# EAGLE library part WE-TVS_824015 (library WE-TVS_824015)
TVS Diode Array WE-TVS, High Speed Series - Low capazity - No leakage current - Low clamping voltage - high ESD voltage protection -- USB 1.0 - 2.0 Double Port -- Ethernet
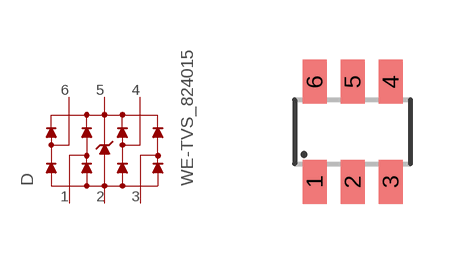
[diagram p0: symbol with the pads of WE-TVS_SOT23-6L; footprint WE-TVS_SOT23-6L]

Designator prefix D

## WE-TVS_824015 (MPN: 824015; OC_FARNELL: 1748615; OC_NEWARK: 34R6122; PACKAGE: SOT23-6L; SUPPLIER: Wuerth Elektronik)  [WE-TVS_SOT23-6L]
1  1  pas
2  GND  pwr
3  2  pas
4  3  pas
5  VDD  pwr
6  4  pas

## Footprint WE-TVS_SOT23-6L (pad centres in mm)
TVS Diode Array WE-TVS
smd 0.6 x 1.1: 1 -0.95,-1.25; 2 0,-1.25; 3 0.95,-1.25; 4 0.95,1.25; 5 0,1.25; 6 -0.95,1.25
